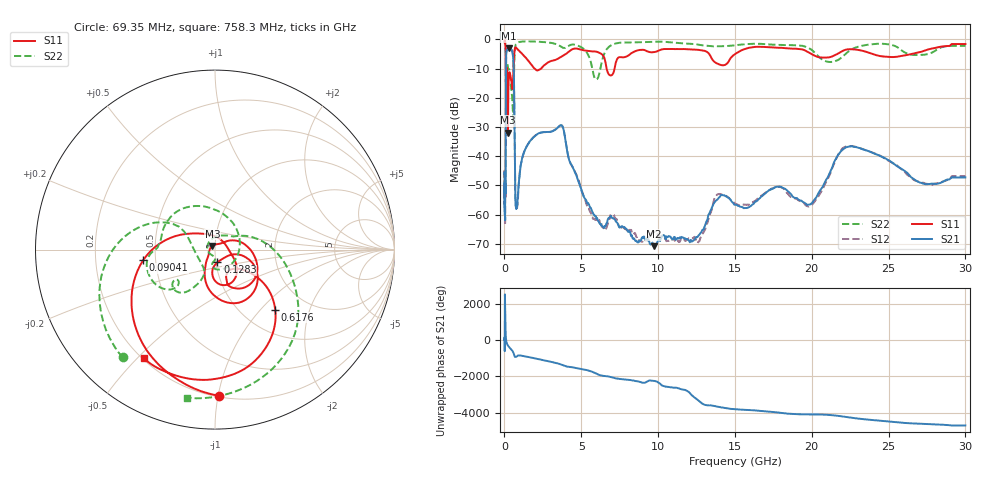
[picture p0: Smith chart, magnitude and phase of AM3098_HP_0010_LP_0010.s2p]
! Date/Time: Thu, Feb 28, 2019 8:32 AM
! Network Analyzer: Agilent Technologies E8364B Rev: A.07.50.67
! Sweep from 0.010 to 30.000 GHz, 1601 Points, Sweep Type: LOG
! Power Supply: 5.022 V, 0.002 A
# Hz S DB R 50
!freq MagS11 AngS11 MagS21 AngS21 MagS12 AngS12 MagS22 AngS22
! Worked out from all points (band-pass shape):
!   1601 points, 10 MHz to 30 GHz, reference 50 ohm
!   highest |S21| = -3.02 dB at 266.5 MHz (marker M1); lowest = -70.8 dB at 9.731 GHz (marker M2)
!   |S21| within 3 dB of the highest: 106.3 MHz to 562.5 MHz (456.3 MHz wide, 136 % of centre)
!   lowest |S11| = -31.9 dB at 228.2 MHz (marker M3), VSWR 1.05, Z = 48.5 + j2.02 ohm
!   |S11| at or under -10 dB: 175.8 MHz to 587.9 MHz (412.1 MHz wide, 108 % of centre); 1.969 GHz to 2.381 GHz (412.6 MHz wide, 19 % of centre); 6.649 GHz to 7.166 GHz (516.7 MHz wide, 7.48 % of centre)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
!   |S22| runs from -29.0 to -0.5 dB; largest |S21 - S12| = 0.01
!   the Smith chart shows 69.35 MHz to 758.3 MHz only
!   S11 on the Smith chart (normalised r, x): 69.35 MHz: 0.21, -1.00; 90.41 MHz: 0.43, -0.06; 128.3 MHz: 1.02, -0.15; 617.6 MHz: 1.40, -1.21; 758.3 MHz: 0.20, -0.52
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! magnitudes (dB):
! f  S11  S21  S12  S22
! 10 MHz  -0.3  -45.9  -45.0  -0.5
! 38.04 MHz  -0.5  -60.9  -60.8  -0.8
! 69.35 MHz  -1.8  -52.3  -53.8  -2.0
! 90.41 MHz  -7.9  -19.6  -19.6  -9.3
! 99.92 MHz  -23.9  -8.0  -8.0  -17.4
! 128.3 MHz  -22.8  -4.1  -4.1  -11.1
! 144.7 MHz  -13.9  -3.6  -3.6  -10.3
! 187.7 MHz  -11.6  -3.4  -3.4  -8.3
! 228.2 MHz  -31.9  -3.1  -3.1  -9.9
! 266.5 MHz  -15.0  -3.0  -3.0  -10.3
! 550.5 MHz  -14.9  -5.4  -5.4  -25.1
! 617.6 MHz  -6.5  -13.3  -13.3  -13.2
! 699.9 MHz  -2.7  -51.9  -52.1  -2.5
! 758.3 MHz  -2.8  -57.8  -57.0  -1.5
! 2.084 GHz  -10.5  -32.6  -32.7  -0.7
! 3.723 GHz  -5.9  -29.4  -29.4  -2.6
! 5.989 GHz  -4.2  -61.5  -61.8  -13.7
! 7.926 GHz  -5.9  -64.9  -65.1  -1.0
! 9.731 GHz  -4.3  -70.8  -65.9  -0.8
! 19.8 GHz  -4.5  -56.5  -57.2  -3.0
! 22.67 GHz  -3.4  -36.7  -36.5  -3.2
! 30 GHz  -1.6  -47.3  -46.8  -2.2
